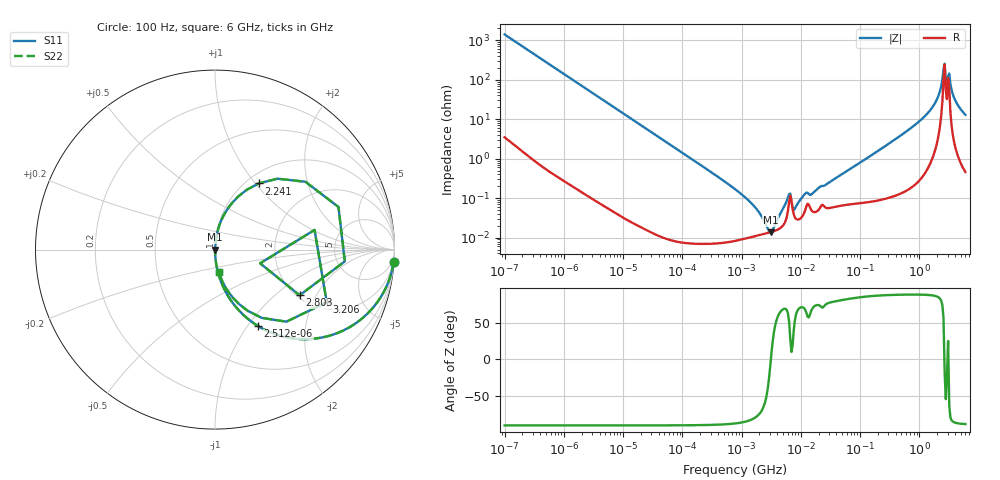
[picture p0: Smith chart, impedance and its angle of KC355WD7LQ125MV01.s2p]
!Murata Part Number: KC355WD7LQ125MV01
!These Parameters are Measured in Series Mode Connection
!Data Generated on Jun 19, 2026
!  o--ll--o
!Port1  Port2
!  o------o
!Operation Temp=25[degC], DC Bias Voltage=0[V]
!Freq. Start=100[Hz] Stop=6[GHz] 401[Steps]
# Hz S RI R 50
!Freq.(Hz) S11(Real) S11(Imag) S21(Real) S21(Imag) S12(Real) S12(Imag) S22(Real) S22(Imag)
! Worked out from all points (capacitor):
!   401 points, 100 Hz to 6 GHz, reference 50 ohm
!   read as one part in series: C = 1.13 uF near 109 Hz
!   lowest |Z| = 13.8 mohm at 3.104 MHz (marker M1)
!   series resonance near 3.122 MHz, so ESL is about 2.3 nH
!   S11 on the Smith chart (normalised r, x): 100 Hz: 1, -28; 2.512 kHz: 1.00, -1.12; 2.241 GHz: 1.14, +1.04; 2.803 GHz: 2.07, -1.48; 3.206 GHz: 2.30, -2.57; 6 GHz: 1.01, -0.26
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100  0.9948 -0.0708  0.00522 0.0708  0.00522 0.0708  0.9948 -0.0708
524  0.8778 -0.3266  0.1222 0.3266  0.1222 0.3266  0.8778 -0.3266
2008  0.3305 -0.4694  0.6695 0.4694  0.6695 0.4694  0.3305 -0.4694
2512  0.2401 -0.4261  0.7599 0.4261  0.7599 0.4261  0.2401 -0.4261
6433  0.0464 -0.2092  0.9536 0.2092  0.9536 0.2092  0.0464 -0.2092
40335  0.00134 -0.035  0.9987 0.035  0.9987 0.035  0.00134 -0.035
774597  8.56e-05 -0.0017  0.9999 0.0017  0.9999 0.0017  8.56e-05 -0.0017
1658239  0.000109 -0.000601  0.9999 0.000601  0.9999 0.000601  0.000109 -0.000601
3103719  0.000138 -5.3e-06  0.9999 5.3e-06  0.9999 5.3e-06  0.000138 -5.3e-06
6075234  0.000485 0.000928  0.9995 -0.000928  0.9995 -0.000928  0.000485 0.000928
7947587  0.000326 0.00044  0.9997 -0.00044  0.9997 -0.00044  0.000326 0.00044
1.189169e7  0.000508 0.00121  0.9995 -0.00121  0.9995 -0.00121  0.000508 0.00121
1.555665e7  0.000471 0.00121  0.9995 -0.00121  0.9995 -0.00121  0.000471 0.00121
3.124326e8  0.00163 0.0245  0.9984 -0.0245  0.9984 -0.0245  0.00163 0.0245
1.251881e9  0.0186 0.1186  0.9814 -0.1186  0.9814 -0.1186  0.0186 0.1186
1.873145e9  0.0812 0.2423  0.9188 -0.2423  0.9188 -0.2423  0.0812 0.2423
2.240541e9  0.2437 0.3686  0.7563 -0.3686  0.7563 -0.3686  0.2437 0.3686
2.450438e9  0.5041 0.378  0.4959 -0.378  0.4959 -0.378  0.5041 0.378
2.802721e9  0.4714 -0.2546  0.5286 0.2546  0.5286 0.2546  0.4714 -0.2546
3.205649e9  0.6226 -0.2933  0.3774 0.2933  0.3774 0.2933  0.6226 -0.2933
4.009986e9  0.1024 -0.271  0.8976 0.271  0.8976 0.271  0.1024 -0.271
6e9  0.0209 -0.1263  0.9791 0.1263  0.9791 0.1263  0.0209 -0.1263
